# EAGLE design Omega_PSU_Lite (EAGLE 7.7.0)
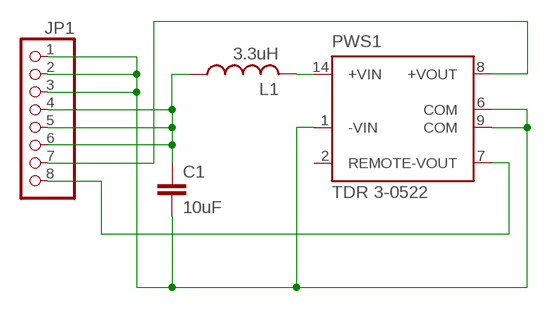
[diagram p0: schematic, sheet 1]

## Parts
C1  10uF  C-EU050-025X075  [C050-025X075]
JP1  PINHD-1X8  [1X08]
L1  3.3uH  L-US0207/12  [0207/12]
PWS1  TDR 3-0522  TDR_30522  [TRACOPOWER3W]

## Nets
GND: C1.2 JP1.1 JP1.2 JP1.3 PWS1.1(-VIN) PWS1.6(COM) PWS1.9(COM)
N$3: L1.2 PWS1.14(+VIN)
VCC: C1.1 JP1.4 JP1.5 JP1.6 L1.1
VDD: JP1.7 PWS1.8(+VOUT)
VSS: JP1.8 PWS1.7(-VOUT)
Unconnected: PWS1.2(REMOTE)

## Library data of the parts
C1 = rcl:C-EU: CAPACITOR, European symbol
JP1 = pinhead:PINHD-1X8: PIN HEADER
L1 = rcl:L-US: INDUCTOR, American symbol
PWS1 = TRACO_TDR:TDR_3: DC/DC-Konverter 3 Watt, 1 x Input, 1 x +- Output Source: https://assets.tracopower.com/20200124074754/TDR3/documents/tdr3-datasheet.pdf

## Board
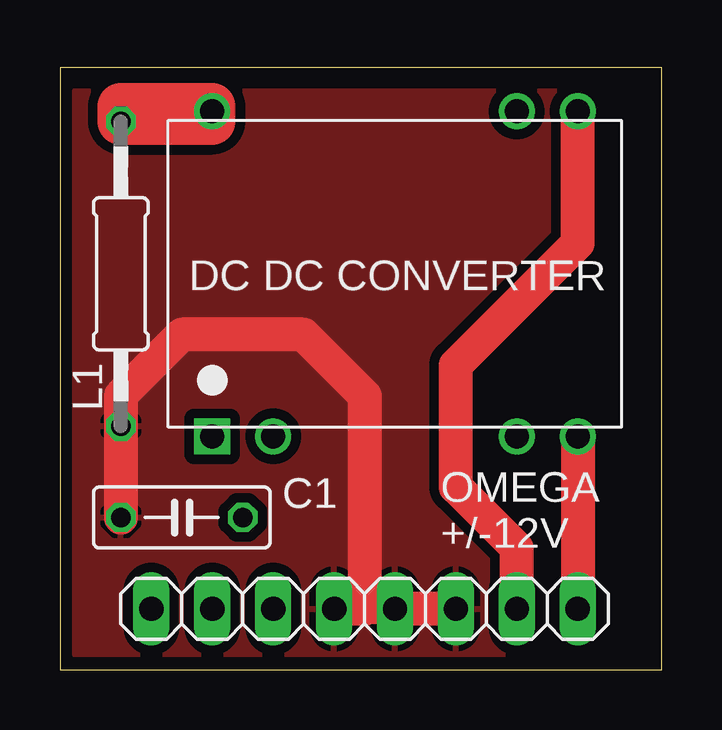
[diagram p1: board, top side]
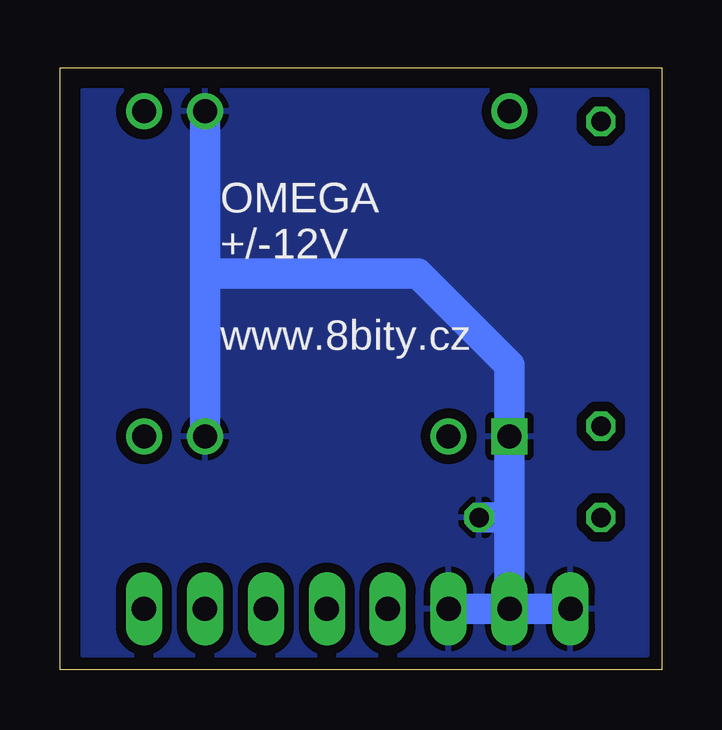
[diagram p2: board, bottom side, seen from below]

Size 25.09 x 25.09 mm. Coordinates in mm from the lower left corner, seen from the top.
Outline: 0,0 25.09,0 25.09,25.09 0,25.09 0,0
Copper layers (1*16): Top 0.0356mm / dielectric 1.5011mm / Bottom 0.0356mm
Design rules "oshpark-2layer": minimum track width 6mil, minimum drill 13mil, track to track 6mil, track to pad 6mil, pad to pad 6mil, via to via 6mil, smd to smd 6mil, copper to edge 15mil, drill to drill 6mil, minimum pad ring 7mil, minimum via ring 7mil, stop-mask expansion 2.5mil, vias tented up to drill 0mil, thermal gap 10mil

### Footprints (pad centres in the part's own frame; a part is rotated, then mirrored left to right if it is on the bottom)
C050-025X075 = drill 0.813 octagon: 1 -2.54,0; 2 2.54,0
1X08 = drill 1.016 long: 1 -8.89,0; 2 -6.35,0; 3 -3.81,0; 4 -1.27,0; 5 1.27,0; 6 3.81,0; 7 6.35,0; 8 8.89,0
0207/12 = drill 0.813 octagon: 1 -6.35,0; 2 6.35,0
TRACOPOWER3W = drill 1 square: 1 -7.62,-6.775 | drill 1: 2 -5.08,-6.775; 6 5.08,-6.775; 7 7.62,-6.775; 8 7.62,6.775; 9 5.08,6.775; 14 -7.62,6.775

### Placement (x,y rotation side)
C1  5.08,6.35 0 top
JP1  12.7,2.54 0 top
L1  2.54,16.51 90 top
PWS1  13.97,16.51 0 top

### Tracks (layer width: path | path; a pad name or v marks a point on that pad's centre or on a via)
GND
  Bottom 1.27: JP1.1 JP1.2 | 6.35,6.35 PWS1.1 6.35,12.7 10.16,16.51 19.05,16.51 | 6.35,6.35 JP1.2 | C1.2 6.35,6.35 | JP1.2 JP1.3 | PWS1.9 19.05,16.51 | 19.05,16.51 PWS1.6
  pour Bottom (isolate 0.406): 0.64,0.64 0.64,24.13 24.13,24.13 24.13,0.64
N$3
  Top 1.93: L1.2 5.92,22.86 PWS1.14 | L1.2 6.35,22.86 6.35,23.5 2.54,23.5 L1.2
VCC
  Top 1.27: JP1.5 12.7,2.54
  Top 1.422: C1.1 L1.1 2.54,11.43 5.08,13.97 10.16,13.97 12.7,11.43 12.7,2.54 JP1.4 | JP1.6 JP1.5
  pour Top (isolate 0.406): 0.64,0.64 0.64,24.13 24.13,24.13 24.13,0.64
VDD
  Top 1.422: JP1.7 19.05,5.08 16.51,7.62 16.51,12.7 21.59,17.78 PWS1.8
VSS
  Top 1.422: PWS1.7 JP1.8

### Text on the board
tNames: OMEGA / +/-12V
bNames: OMEGA / +/-12V / / www.8bity.cz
